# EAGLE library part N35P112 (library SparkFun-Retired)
Hall-effect based I2C analog mini-joystick with button
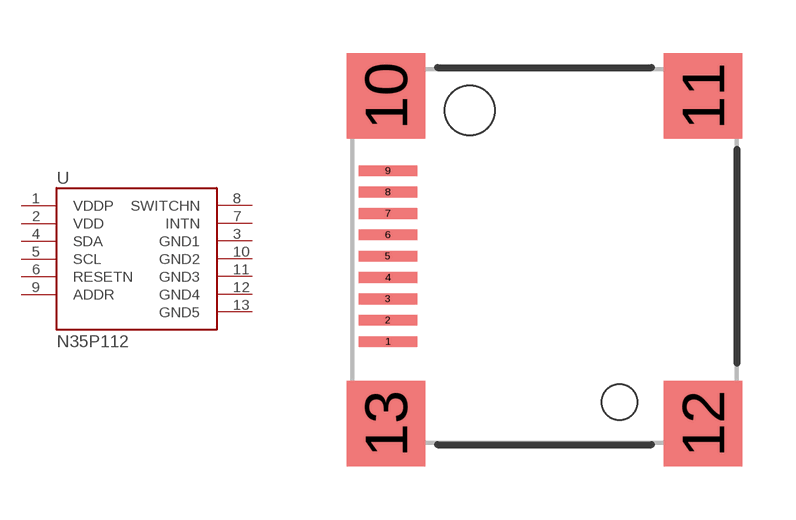
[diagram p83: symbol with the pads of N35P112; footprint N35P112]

Designator prefix U

## N35P112 (PROD_ID: SWCH-10635)  [N35P112]
1  VDDP
2  VDD
3  GND1
4  SDA
5  SCL
6  RESETN
7  INTN
8  SWITCHN
9  ADDR
10  GND2
11  GND3
12  GND4
13  GND5

## Footprint N35P112 (pad centres in mm)
smd 1.65 x 0.3: 1 -4.4,-2.4; 2 -4.4,-1.8; 3 -4.4,-1.2; 4 -4.4,-0.6; 5 -4.4,0; 6 -4.4,0.6; 7 -4.4,1.2; 8 -4.4,1.8; 9 -4.4,2.4
smd 2.2 x 2.4: 10 -4.45,4.5; 11 4.45,4.5; 12 4.45,-4.7; 13 -4.45,-4.7
hole 1.4 at -2.1,4.1
hole 1 at 2.1,-4.1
